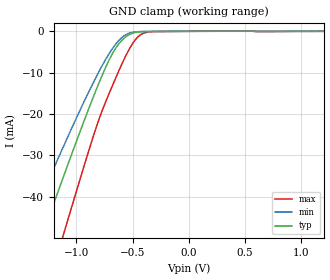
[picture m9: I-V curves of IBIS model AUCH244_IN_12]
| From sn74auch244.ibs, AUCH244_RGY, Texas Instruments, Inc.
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[Model]   AUCH244_IN_12
Model_type  Input
Vinl=0.385
Vinh=0.845
| variable   typ   min   max
C_comp   2.56pF   2.12pF   2.86pF
[Temperature Range]   40   100   -40
| Ambient temperature   25   85   -40
[Voltage range]   1.2   1.1   1.3
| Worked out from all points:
|   GND clamp passes 1 mA (typ) near -0.54 V on its own axis
[GND Clamp]
| AUCH244_IN_12
|   Voltage   I(typ)   I(min)   I(max)
-3.6V     -227.9mA   -191.3mA   -273.5mA
-1.47V    -62.2mA    -50.04mA   -81.61mA
-1.425V   -58.74mA   -47.18mA   -77.5mA
-1.295V   -48.79mA   -38.98mA   -65.64mA
-1.13V    -36.31mA   -28.8mA    -50.57mA
-1.09V    -33.32mA   -26.37mA   -46.92mA
-835mV    -14.93mA   -11.66mA   -24.21mA
-700mV    -6.485mA   -5.058mA   -14.49mA
-575mV    -1.666mA   -1.082mA   -6.759mA
-440mV    -145.9uA   -77.53uA   -1.064mA
-300mV    -34.28uA   -20.8uA    -73.64uA
1.2V      141.8pA    532.6nA    24.7pA
